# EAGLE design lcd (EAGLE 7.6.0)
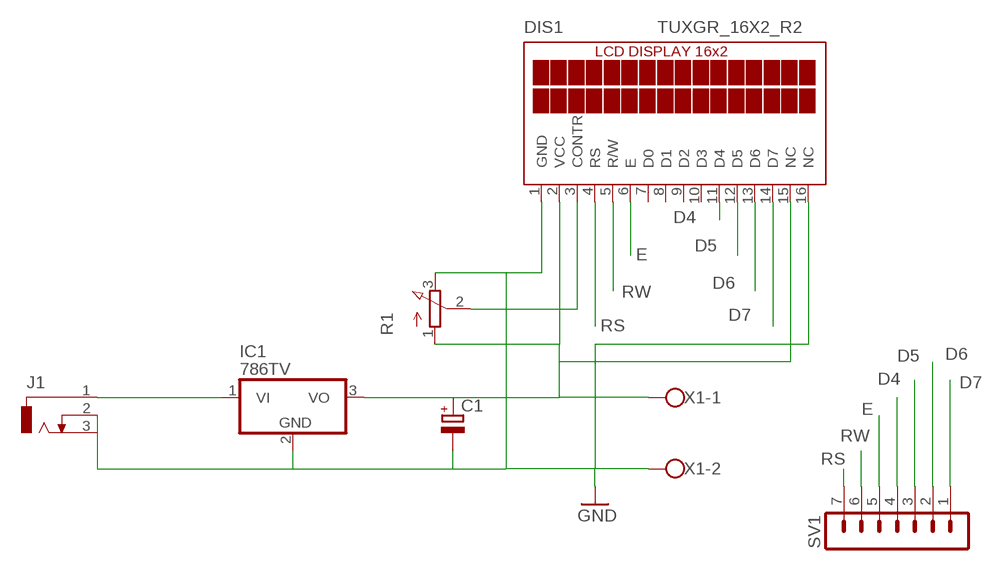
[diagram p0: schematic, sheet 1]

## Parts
C1  CPOL-EUE2,5-6E  [E2,5-6E]
DIS1  TUXGR_16X2_R2  [TUXGR_16X2_R2]
IC1  786TV  [TO220V]
J1  DCJ0303  [DCJ0303]
R1  3RP/1610N  [3RP/1610N]
SV1  MA07-1  [MA07-1]
X1  W237-102  [W237-102]

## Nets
D4: DIS1.11(D4) SV1.4
D5: DIS1.12(D5) SV1.3
D6: DIS1.13(D6) SV1.2
D7: DIS1.14(D7) SV1.1
E: DIS1.6(E) SV1.5
GND: C1.- DIS1.1(GND) DIS1.16(NC) IC1.2(GND) J1.2 J1.3 R1.3(E) X1.2
N$1: IC1.1(VI) J1.1
N$3: C1.+ DIS1.2(VCC) DIS1.15(NC) IC1.3(VO) R1.1(A) X1.1
N$6: DIS1.3(CONTR) R1.2(S)
RS: DIS1.4(RS) SV1.7
RW: DIS1.5(R/W) SV1.6
Unconnected: DIS1.7(D0) DIS1.8(D1) DIS1.9(D2) DIS1.10(D3)

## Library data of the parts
C1 = rcl:CPOL-EU: POLARIZED CAPACITOR, European symbol
DIS1 = display-lcd:TUXGR_16X2_R2: Tuxgraphics LCD display 16x2 characters reflective, without background light Source: tuxgr_12x2_r2.pdf; OC_FARNELL: unknown; OC_NEWARK: unknown
IC1 = linear:78*: Positive VOLTAGE REGULATOR Source: http://cache.national.com/ds/LM/LM78L05.pdf http://www.fairchildsemi.com/ds/LM/LM7805.pdf
J1 = con-jack:DCJ0303: DC POWER JACK Source: DCJ0303.pdf; OC_FARNELL: unknown; OC_NEWARK: unknown
R1 = pot:3RP/1610N: 16mm Potentiometer one level Source: http://www.alphapotentiometers.net/html/16mm_pot_2.html
SV1 = con-lstb:MA07-1: PIN HEADER; OC_FARNELL: unknown; OC_NEWARK: unknown
X1 = con-wago-500:W237-102: WAGO SCREW CLAMP; MPN: 237-102; OC_FARNELL: unknown; OC_NEWARK: 70K9898

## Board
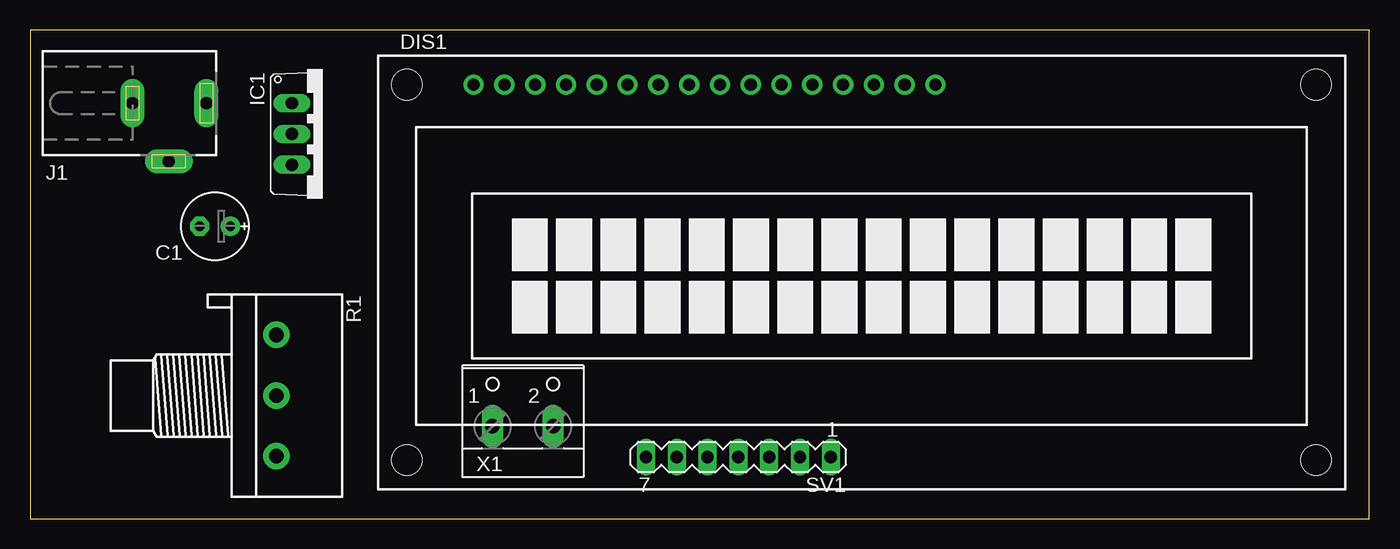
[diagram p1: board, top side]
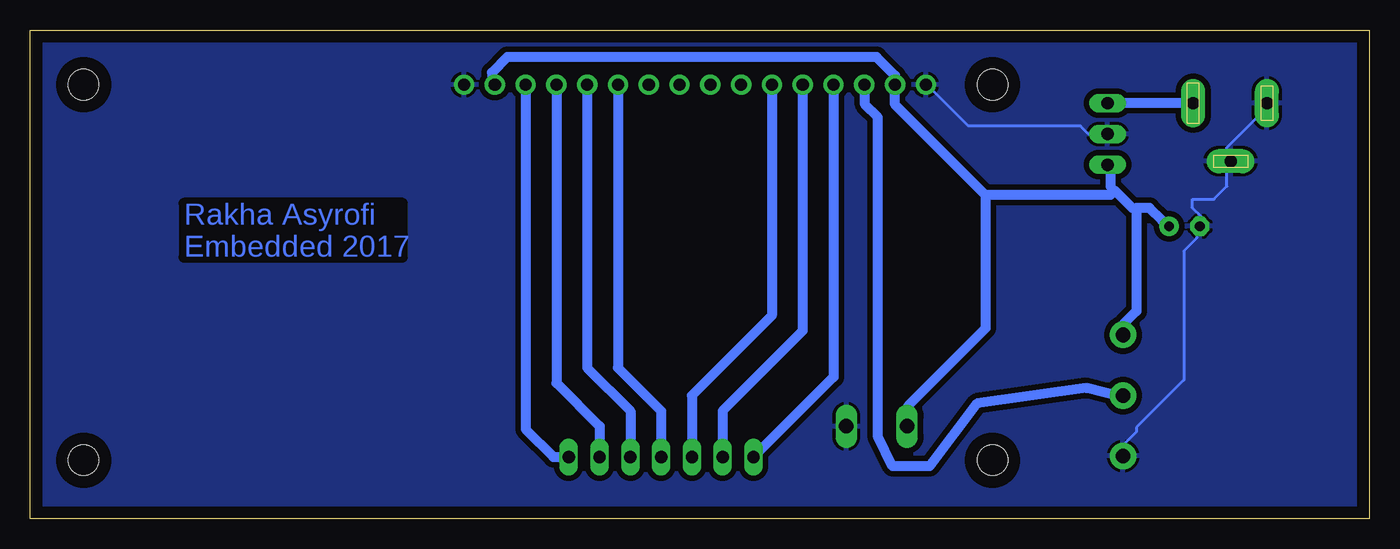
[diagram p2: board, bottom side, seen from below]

Size 110.47 x 40.31 mm. Coordinates in mm from the lower left corner, seen from the top.
Outline: 0,0 110.47,0 110.47,40.31 0,40.31 0,0
Copper layers (1*16): Top 0.035mm / dielectric 1.5mm / Bottom 0.035mm
Design rules "default *": minimum track width 10mil, minimum drill 24mil, track to track 18mil, track to pad 18mil, pad to pad 18mil, via to via 18mil, smd to smd 8mil, copper to edge 40mil, drill to drill 8mil, minimum pad ring 10mil, minimum via ring 8mil, stop-mask expansion 4mil, vias tented up to drill 0mil, thermal gap 10mil

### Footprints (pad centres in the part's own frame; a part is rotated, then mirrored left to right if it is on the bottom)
E2,5-6E = drill 0.813 pad 1.575: + -1.27,0 | drill 0.813 pad 1.575 octagon: - 1.27,0
TUXGR_16X2_R2 = drill 1 pad 1.676: 1 -32,15.5; 2 -29.46,15.5; 3 -26.92,15.5; 4 -24.38,15.5; 5 -21.84,15.5; 6 -19.3,15.5; 7 -16.76,15.5; 8 -14.22,15.5; 9 -11.68,15.5; 10 -9.14,15.5; 11 -6.6,15.5; 12 -4.06,15.5; 13 -1.52,15.5; 14 1.02,15.5; 15 3.56,15.5; 16 6.1,15.5 | hole 2.5: -37.5,-15.5; 37.5,-15.5; -37.5,15.5; 37.5,15.5
TO220V = drill 1.016 long: 1 -2.54,-2.54; 2 0,-2.54; 3 2.54,-2.54
DCJ0303 = drill 1 pad 2 long: 1 0,3.1; 2 4.8,0; 3 0,-3
3RP/1610N = drill 1.2 pad 2.184: 1 -5,0; 2 0,0; 3 5,0
MA07-1 = drill 1.016 long: 1 -7.62,0; 2 -5.08,0; 3 -2.54,0; 4 0,0; 5 2.54,0; 6 5.08,0; 7 7.62,0
W237-102 = drill 1.194 long: 1 -2.5,-1.27; 2 2.5,-1.27

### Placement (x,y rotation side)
C1  15.24,24.13 180 top
DIS1  68.58,20.32 0 top
IC1  24.13,31.75 270 top
J1  11.43,34.29 270 top
R1  20.32,10.16 270 top
SV1  58.42,5.08 180 top
X1  40.64,8.89 0 top

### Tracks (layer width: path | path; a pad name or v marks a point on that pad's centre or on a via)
D4
  Bottom 0.813: DIS1.11 61.98,12.45 58.42,8.89 SV1.4
D5
  Bottom 0.813: DIS1.12 64.52,12.45 60.96,8.89 SV1.3
D6
  Bottom 0.813: DIS1.13 67.06,11.18 63.5,7.62 SV1.2
D7
  Bottom 0.813: DIS1.14 69.6,7.37 67.31,5.08 SV1.1
E
  Bottom 0.813: DIS1.6 49.28,16.76 55.88,10.16 SV1.5
GND
  Bottom 0.254: 23.11,31.7 23.82,32.41 33.07,32.41 36.27,35.61 DIS1.1 | J1.3 8.53,34.19 9.25,33.48 9.25,33.12 11.73,30.63 11.73,29.57 J1.2 11.73,29.21 11.73,27.43 12.8,26.37 14.58,26.37 14.58,25.65 13.87,24.94 13.87,24.23 C1.- 14.22,23.88 14.22,23.17 15.29,22.1 15.29,11.43 19.2,7.52 19.2,7.16 20.27,6.1 20.27,5.39 R1.3
  pour Bottom: 0,40.64 110.49,40.64 110.49,0 0,0
N$1
  Bottom 0.813: J1.1 IC1.1
N$3
  Bottom 0.254: 21.34,27.43 20.98,27.08 21.34,26.72 | 19.2,25.65 19.56,25.65 | 17.07,24.59 16.71,24.59 16.36,24.23 C1.+ | 21.34,29.21 IC1.3 | 39.12,36.68 39.12,35.97 DIS1.2 | 38.05,7.87 X1.1 | 20.27,15.34 R1.1
  Bottom 0.813: 21.34,27.43 21.34,29.21 | 19.56,25.65 20.98,27.08 | 17.07,24.59 18.14,25.65 19.2,25.65 19.2,17.12 20.27,16.05 20.27,15.34 | 31.65,26.72 39.12,34.19 39.12,35.61 DIS1.2 39.12,36.58 40.64,38.1 71.12,38.1 72.39,36.83 72.39,36.07 DIS1.15 | 21.34,26.72 31.65,26.72 | 38.05,7.87 38.05,9.3 31.65,15.7 31.65,26.72
N$6
  Bottom 0.254: 41.6,35.61 DIS1.3 | 20.27,10.01 R1.2
  Bottom 0.813: 41.6,35.61 41.6,34.19 40.54,33.12 40.54,6.81 39.32,4.32 36.27,4.32 32.36,9.5 23.32,10.77 20.27,10.01
RS
  Bottom 0.813: DIS1.4 44.2,11.68 SV1.7
RW
  Bottom 0.813: DIS1.5 46.74,15.49 53.34,8.89 SV1.6

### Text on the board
Bottom: Rakha Asyrofi / Embedded 2017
